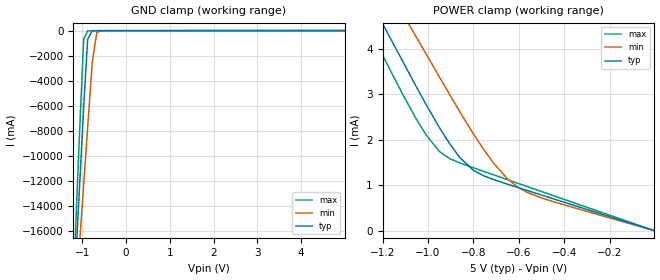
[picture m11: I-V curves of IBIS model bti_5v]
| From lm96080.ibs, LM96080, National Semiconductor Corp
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[Model] bti_5v
Model_type Input
Vinh = 2.0V
Vinl = 0.8V
C_comp   2.30pF   2.10pF   2.51pF
[Voltage Range]   5.0V   4.5V   5.5V
[Temperature Range]   25.0   125.0   -40.0
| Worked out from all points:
|   POWER clamp passes 1 mA (typ) near -0.63 V on its own axis
[GND Clamp]
-5V       -276.6A    -215.3A    -345.2A
-1.175V   -20.24A    -22.93A    -18.03A
-1.07V    -13.15A    -17.6A     -9.004A
-965mV    -6.114A    -12.29A    -679.3mA
-875mV    -701.3mA   -7.767A    -25.8mA
-770mV    -25.15mA   -2.535A    -9.784mA
-665mV    -8.026mA   -145.6mA   -7.787mA
-560mV    -6.698mA   -13.9mA    -7.529mA
-470mV    -6.517mA   -6.5mA     -7.432mA
4.99V     -15.52uA   0A         -849.8uA
[POWER Clamp]
-5V       39.99mA    38.08mA    41.34mA
-1.265V   5.154mA    6.081mA    4.498mA
-1.205V   4.594mA    5.567mA    3.906mA
-1.16V    4.175mA    5.182mA    3.463mA
-1.115V   3.755mA    4.796mA    3.031mA
-1.055V   3.196mA    4.282mA    2.485mA
-950mV    2.268mA    3.383mA    1.742mA
-860mV    1.61mA     2.616mA    1.491mA
-800mV    1.329mA    2.13mA     1.384mA
-710mV    1.123mA    1.481mA    1.227mA
-605mV    952.6uA    959.7uA    1.045mA
-5mV      7.768uA    7.041uA    8.565uA
